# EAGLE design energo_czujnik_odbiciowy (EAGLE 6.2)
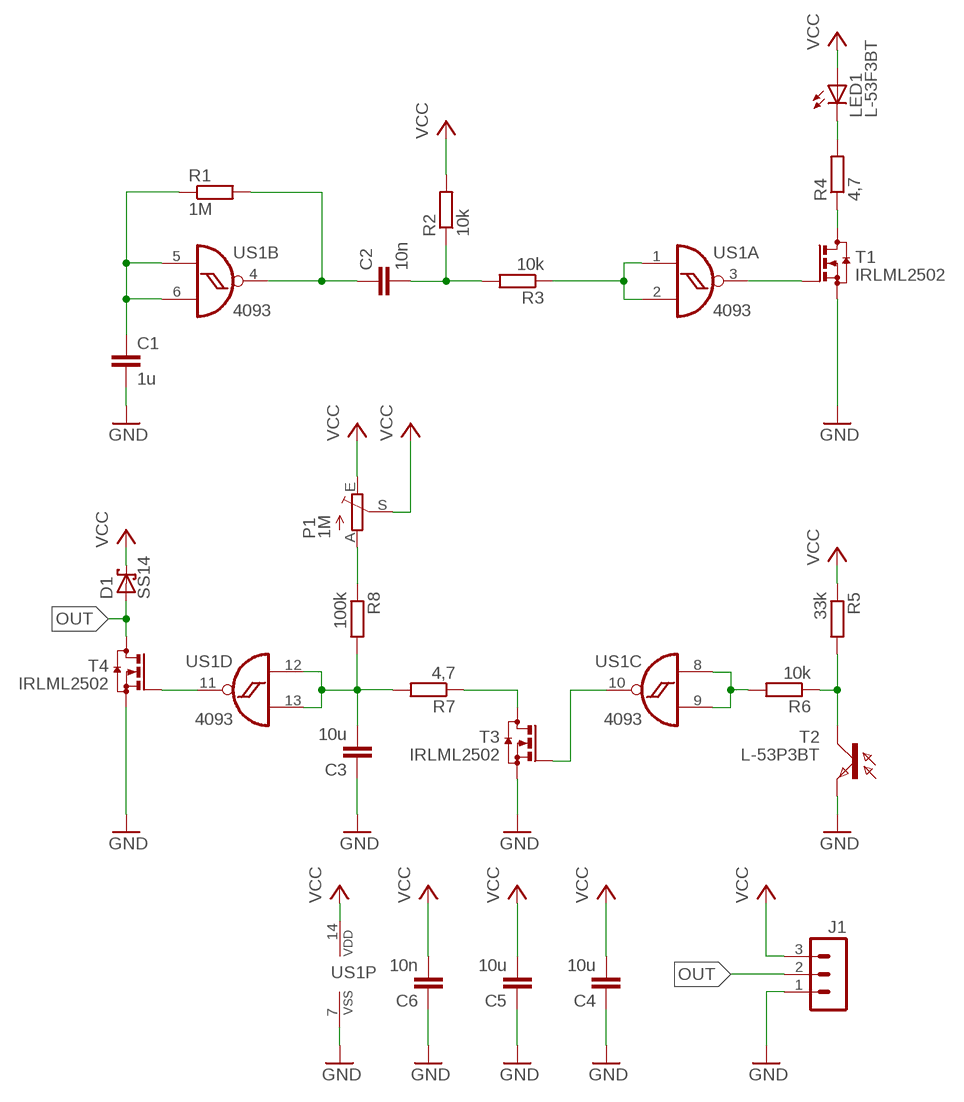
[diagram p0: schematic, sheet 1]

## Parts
C1  1u  C-EUC0805  [C0805]
C2  10n  C-EUC0805  [C0805]
C3  10u  C-EUC0805  [C0805]
C4  10u  C-EUC0805  [C0805]
C5  10u  C-EUC0805  [C0805]
C6  10n  C-EUC0805  [C0805]
D1  SS14  SCHOTTKY-DIODESMD  [SMB]
J1  MA03-1  [MA03-1]
LED1  L-53F3BT  LEDLD260  [LD260]
P1  1M  TRIM_EU-CA6V  [CA6V]
R1  1M  R-EU_M0805  [M0805]
R2  10k  R-EU_M0805  [M0805]
R3  10k  R-EU_M0805  [M0805]
R4  4,7  R-EU_M1206  [M1206]
R5  33k  R-EU_M0805  [M0805]
R6  10k  R-EU_M0805  [M0805]
R7  4,7  R-EU_M1206  [M1206]
R8  100k  R-EU_M0805  [M0805]
T1  IRLML2502  BSS123  [SOT23]
T2  L-53P3BT  BPX81  [BPX81]
T3  IRLML2502  BSS123  [SOT23]
T4  IRLML2502  BSS123  [SOT23]
US1  4093  4093D  [SO14]

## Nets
GND: C1.2 C3.1 C4.1 C5.1 C6.1 J1.1 T1.2(S) T2.E T3.2(S) T4.2(S) US1.7(P:VSS)
N$1: C1.1 R1.1 US1.5(B:I0) US1.6(B:I1)
N$2: C2.1 R1.2 US1.4(B:O)
N$3: R3.1 US1.1(A:I0) US1.2(A:I1)
N$4: C2.2 R2.1 R3.2
N$5: T1.1(G) US1.3(A:O)
N$6: R4.1 T1.3(D)
N$7: LED1.K(C) R4.2
N$8: R5.2 R6.1 T2.C
N$9: C3.2 R7.2 R8.2 US1.12(D:I0) US1.13(D:I1)
N$10: P1.A R8.1
N$11: T3.1(G) US1.10(C:O)
N$12: R7.1 T3.3(D)
N$13: T4.1(G) US1.11(D:O)
N$14: R6.2 US1.8(C:I0) US1.9(C:I1)
OUT: D1.A J1.2 T4.3(D)
VCC: C4.2 C5.2 C6.2 D1.C J1.3 LED1.A P1.E P1.S R2.2 R5.1 US1.14(P:VDD)

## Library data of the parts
C1-C6 = rcl:C-EU: CAPACITOR, European symbol
D1 = diode:SCHOTTKY-DIODE: Schottky Diode
J1 = con-lstb:MA03-1: PIN HEADER; OC_FARNELL: unknown; OC_NEWARK: unknown
LED1 = led:LED: LED
P1 = pot:TRIM_EU-: POTENTIOMETER
R1-R8 = rcl:R-EU_: RESISTOR, European symbol
T1 T3 T4 = transistor-small-signal:BSS123: N-CHANNEL MOS FET
T2 = opto-trans-siemens:BPX81: PHOTO TRANSISTOR; OC_FARNELL: unknown; OC_NEWARK: unknown
US1 = 40xx:4093: Quad 2-input NAND schmitt trigger

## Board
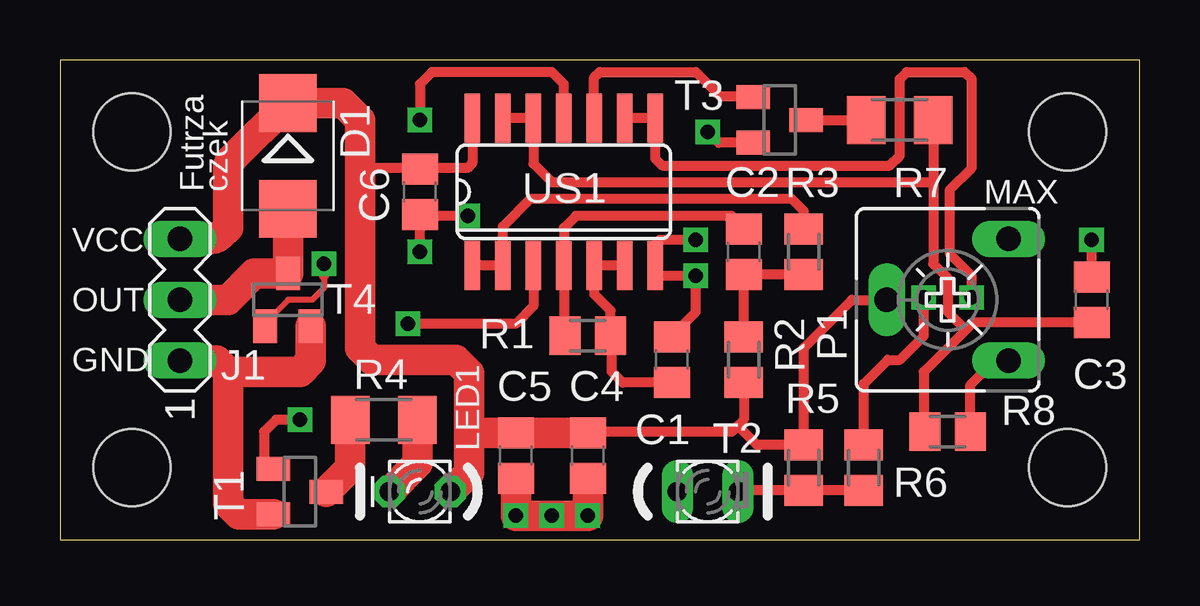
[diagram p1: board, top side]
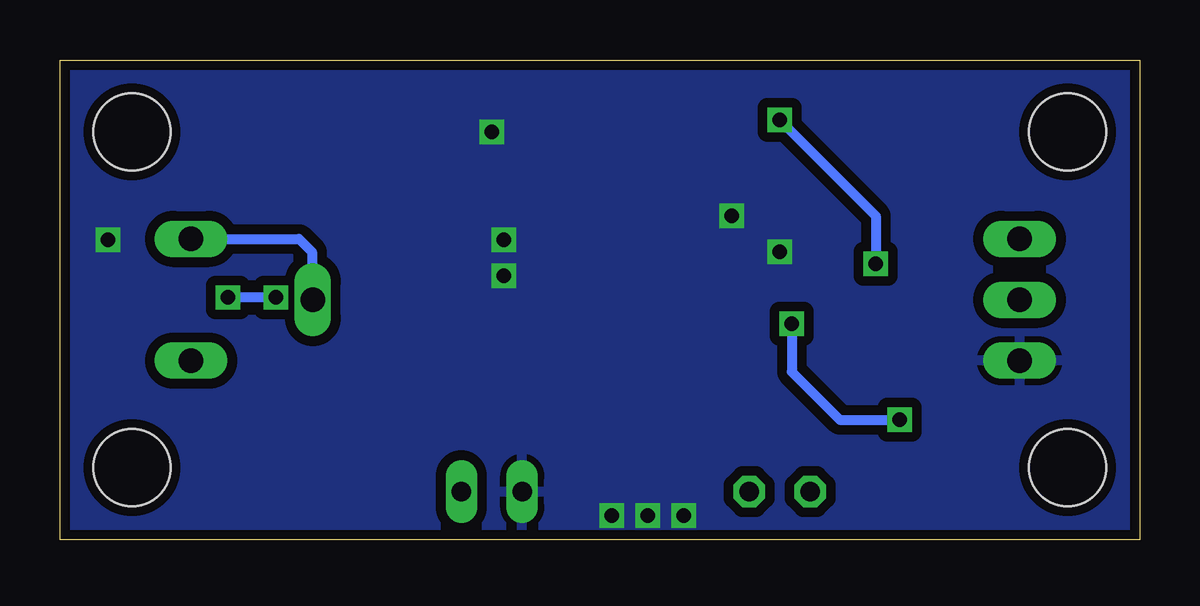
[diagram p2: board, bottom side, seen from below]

Size 45 x 20 mm. Coordinates in mm from the lower left corner, seen from the top.
Outline: 0,0 45,0 45,20 0,20 0,0
Copper layers (1*16): Top 0.035mm / dielectric 1.5mm / Bottom 0.035mm
Design rules: minimum track width 10mil, minimum drill 23mil, track to track 8mil, track to pad 8mil, pad to pad 8mil, via to via 8mil, smd to smd 8mil, copper to edge 10mil, drill to drill 8mil, minimum pad ring 10mil, minimum via ring 8mil, stop-mask expansion 4mil, vias tented up to drill 0mil, thermal gap 10mil
Holes 3.2 mm at 3,3 3,17 42,3 42,17

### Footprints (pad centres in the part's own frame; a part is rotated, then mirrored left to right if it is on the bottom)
C0805 = smd 1.3 x 1.5: 1 -0.95,0; 2 0.95,0
SMB = smd 2.4 x 2.4: A 2.2,0; C -2.2,0
MA03-1 = drill 1.016 long: 1 -2.54,0; 2 0,0; 3 2.54,0
LD260 = drill 0.813 octagon: A -1.27,0; K 1.27,0
CA6V = drill 1.016 long: A -2.54,-2.54; E 2.54,-2.54; S 0,2.54
M0805 = smd 1.3 x 1.6: 1 -0.95,0; 2 0.95,0
M1206 = smd 1.6 x 2: 1 -1.4,0; 2 1.4,0
SOT23 = smd 1 x 1.4: 1 -0.95,-1.1; 2 0.95,-1.1; 3 0,1.1
BPX81 = drill 0.813 long: C 1.27,0; E -1.27,0
SO14 = smd 0.66 x 2.032: 1 -3.81,-3.073; 2 -2.54,-3.073; 3 -1.27,-3.073; 4 0,-3.073; 5 1.27,-3.073; 6 2.54,-3.073; 7 3.81,-3.073; 8 3.81,3.073; 9 2.54,3.073; 10 1.27,3.073; 11 0,3.073; 12 -1.27,3.073; 13 -2.54,3.073; 14 -3.81,3.073

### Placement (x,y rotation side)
C1  25.5,7.5 90 top
C2  28.5,12 270 top
C3  43,10 270 top
C4  22,3.5 90 top
C5  19,3.5 90 top
C6  15,14.5 90 top
D1  9.5,16 270 top
J1  5,10 90 top
LED1  15,2 180 top
P1  37,10 90 top
R1  22,8.5 180 top
R2  28.5,7.5 270 top
R3  31,12 270 top
R4  13.5,5 0 top
R5  31,3 270 top
R6  33.5,3 90 top
R7  35,17.5 0 top
R8  37,4.5 180 top
T1  10,2 270 top
T2  27,2 0 top
T3  30,17.5 270 top
T4  9.5,10 0 top
US1  21,14.5 0 top

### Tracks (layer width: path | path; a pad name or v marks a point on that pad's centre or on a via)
GND  (via drill 0.6)
  Top 0.406: 14.95,13.5 C6.1 | v15,12 C6.1 | v26.5,12.5 25,12.5 24.81,12.31 US1.7 24.81,11.19 25,11 v26.5,11 26.5,9.5 25.5,8.5 C1.2 | v17,13.5 15.05,13.5 C6.1 | C3.1 v43,12.5 | T3.2 27.45,16.55 v27,17
  Top 1.27: J1.1 6.54,7.46 7,7 | 7,7 10,7 10.45,7.45 T4.2 | T1.2 7.45,1.05 7,1.5 7,7 | C5.1 v19,1 v20.5,1 v22,1 C4.1
  pour Bottom (isolate 0.406): 0,20 45,20 45,0 0,0
N$1
  Top 0.406: US1.6 US1.5 22.27,10.23 22.95,9.55 R1.1 23,8.45 23,7 23.45,6.55 C1.1
N$2
  Top 0.406: R1.2 21,8.55 US1.4 21,13 21.5,13.5 28,13.5 28.5,13 C2.1
N$3
  Top 0.406: US1.1 US1.2 18.46,13.06 19.6,14.2 30.5,14.2 31,13.7 R3.1
N$4
  Top 0.406: R2.1 C2.2 R3.2
N$5  (via drill 0.6)
  Top 0.406: US1.3 19.73,9.73 19,9 v14.5,9 | v10,5 9,5 8.5,4.5 8.5,3.35 T1.1
  Bottom 0.406: v14.5,9 14.5,7 12.5,5 v10,5
N$6
  Top 1.27: R4.1 12.1,3 T1.3
N$7
  Top 1.27: R4.2 14.9,3.17 LED1.K
N$8
  Top 0.406: T2.C 28.32,2.05 R5.2 R6.1
N$9
  Top 0.406: US1.13 US1.12 19.73,15.67 20.5,14.9 36.4,14.9 | C3.2 38.05,9.05 37.75,8.75 | 37.75,8.75 36,7 36,4.55 R8.2 | R7.2 36.4,14.9 | 36.4,14.9 36.4,11.5 37,10.9 37,9.5 37.75,8.75
N$10
  Top 0.406: R8.1 37.95,6.45 39,7.5 39.5,7.5 P1.A
N$11
  Top 0.406: US1.10 22.27,19.27 22.5,19.5 26.5,19.5 27.5,18.5 28.85,18.5 T3.1
N$12
  Top 0.406: T3.3 R7.1
N$13  (via drill 0.6)
  Top 0.254: 11,11 11,10.5 10.5,10 9.5,10 8.55,9.05 T4.1
  Top 0.406: US1.11 21,19 20.5,19.5 15.5,19.5 15,19 v15,17.5 | v11,11.5 11,11
  Bottom 0.406: v15,17.5 11,13.5 v11,11.5
N$14  (via drill 0.6)
  Top 0.406: US1.9 US1.8 24.81,15.89 25.1,15.6 34.6,15.6 35,16 35,19.2 35.3,19.5 37.7,19.5 38,19.2 38,15.5 37.1,14.6 37.1,11.9 38,11 v38,10.1 | R6.2 33.5,6.5 34.5,7.5 35,7.5 36,8.5 v36,10.1
  Bottom 0.406: v36,10.1 v38,10.1
OUT
  Top 1.27: D1.A T4.3 8.1,11.1 7,10 J1.2
VCC
  Top 0.406: US1.14 17.19,15.69 17,15.5 15.05,15.5 | 15.05,15.5 C6.2 | 15.05,15.5 12.5,15.5 | R2.2 28.5,5 28.25,4.75 | 28.25,4.75 28,4.5 22.05,4.5 C4.2 | 28.25,4.75 29.05,3.95 R5.1 31,8 33,10 P1.S
  Top 1.27: J1.3 6.28,12.54 arc45 6.73,12.73 7,13 7,15.44 arc-45 7.19,15.89 D1.C 11.8,18.2 12.5,17.5 12.5,15.5 12.5,8 13,7.5 16.5,7.5 17.05,6.95 17.05,4.45 | C4.2 C5.2 17.05,4.45 | 17.05,4.45 17.05,2.78 LED1.A
  Bottom 0.406: P1.E 35.04,12.54 34.5,12 34.5,10.04 P1.S

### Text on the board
tPlace: Futrza | czek | MAX | VCC | OUT | GND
